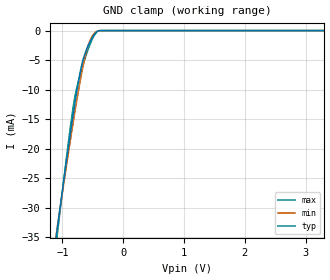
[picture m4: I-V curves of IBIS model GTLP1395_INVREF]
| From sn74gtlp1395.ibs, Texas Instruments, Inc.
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[Model]   GTLP1395_INVREF
Model_type  Input
Vinl = 0.8
Vinh = 2.0
| variable   typ   min   max
C_comp   4.41pF   3.19pF   5.26pF
[Temperature Range]   40   100   -40
| Ambient temperature   25   85   -40
[Voltage range]   3.3   3.15   3.45
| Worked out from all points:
|   GND clamp passes 1 mA (typ) near -0.50 V on its own axis
[GND Clamp]
| GTLP1395_INVREF
|   Voltage   I(typ)   I(min)   I(max)
-5.5V     -409.1mA   -373.4mA   -463.2mA
-1.09V    -33.98mA   -33.73mA   -35.08mA
-1.05V    -30.89mA   -30.92mA   -31.55mA
-865mV    -17.11mA   -18.32mA   -15.97mA
-825mV    -14.31mA   -15.72mA   -13.07mA
-785mV    -11.64mA   -13.19mA   -10.69mA
-730mV    -8.275mA   -9.853mA   -8.288mA
-685mV    -5.971mA   -7.314mA   -6.643mA
-600mV    -3.108mA   -3.33mA    -3.872mA
-525mV    -1.491mA   -1.22mA    -1.843mA
-430mV    -176.8uA   -116.5uA   -183.5uA
3.3V      290.7pA    954.4pA    1.973nA
